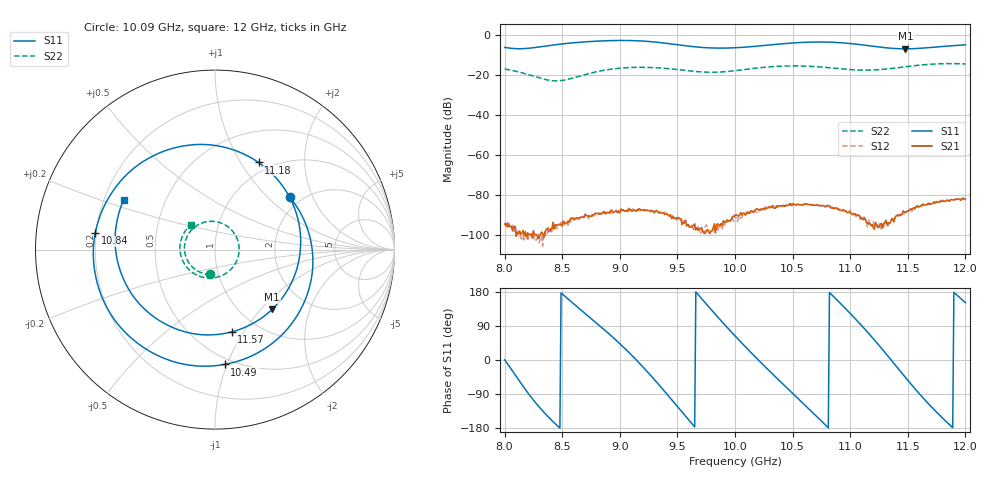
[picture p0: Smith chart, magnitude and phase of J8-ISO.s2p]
!Keysight Technologies,N5234A,MY52241180,A.10.60.03
!Date: Tuesday, May 30, 2023 15:27:16
!Correction: S11(Full 2 Port(1,2))
!S21(Full 2 Port(1,2))
!S12(Full 2 Port(1,2))
!S22(Full 2 Port(1,2))
!S2P File: Measurements: S11, S21, S12, S22:
# Hz S  dB  R 50
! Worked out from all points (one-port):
!   401 points, 8 GHz to 12 GHz, reference 50 ohm
!   lowest |S11| = -6.7 dB at 11.48 GHz (marker M1), VSWR 2.71, Z = 68.6 - j57.9 ohm
!   |S11| at or under -10 dB: nowhere
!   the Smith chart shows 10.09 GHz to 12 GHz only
!   S11 on the Smith chart (normalised r, x): 10.09 GHz: 1.75, +1.37; 10.49 GHz: 0.45, -0.98; 10.84 GHz: 0.20, +0.07; 11.18 GHz: 0.87, +1.20; 11.57 GHz: 0.76, -0.89; 12 GHz: 0.28, +0.24
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8e9  -6.06 0.7  -94.44 155.0  -94.26 136.6  -16.88 119.5
8.27e9  -6.05 -113.2  -99.87 134.0  -102.57 141.0  -20.77 51.7
8.47e9  -4.48 -177.0  -94.62 137.0  -94.82 132.8  -22.74 -25.9
8.67e9  -3.36 130.1  -90.95 94.2  -91.62 94.9  -20.05 -97.7
8.89e9  -2.67 73.4  -88.69 39.1  -88.96 43.4  -17.22 -152.4
9.09e9  -2.59 16.7  -87.33 -12.2  -86.85 -11.6  -16.09 165.1
9.34e9  -3.53 -65.5  -88.98 -74.0  -88.39 -78.8  -16.29 111.3
9.64e9  -5.66 -173.0  -95.16 -131.1  -98.11 -142.6  -17.98 34.8
9.83e9  -6.35 120.3  -98.72 -109.9  -98.97 -112.8  -18.44 -23.5
1e10  -6.19 63.6  -90.17 -132.8  -90.49 -126.5  -17.68 -75.3
1.009e10  -5.88 34.9  -90.06 -146.7  -89.74 -148.9  -17.05 -100.4
1.028e10  -4.91 -23.3  -86.58 168.7  -86.48 169.9  -15.84 -148.1
1.049e10  -3.85 -85.1  -85.23 115.1  -84.43 119.6  -15.30 163.8
1.067e10  -3.35 -137.6  -84.94 68.8  -84.92 68.7  -15.56 122.6
1.084e10  -3.43 172.2  -86.58 24.9  -85.97 25.3  -16.30 80.9
1.102e10  -4.20 116.6  -89.80 -12.8  -88.64 -21.6  -17.19 30.9
1.118e10  -5.31 63.4  -95.15 -20.4  -95.39 -29.6  -17.38 -18.2
1.134e10  -6.37 5.9  -94.16 -5.0  -94.15 -11.4  -16.68 -66.7
1.148e10  -6.73 -46.2  -88.45 -15.1  -88.48 -20.3  -15.69 -105.3
1.157e10  -6.60 -78.6  -85.66 -43.0  -86.17 -41.3  -15.09 -127.9
1.181e10  -5.53 -155.6  -83.02 -96.3  -82.89 -92.9  -14.16 176.5
1.2e10  -4.73 151.3  -81.82 -143.1  -82.31 -143.4  -14.33 134.3
